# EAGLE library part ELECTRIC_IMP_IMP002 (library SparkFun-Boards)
Electric Imp Module imp002 Datasheet SparkFun Products SparkFun Electric Imp imp002 Breakout (BOB-12958)
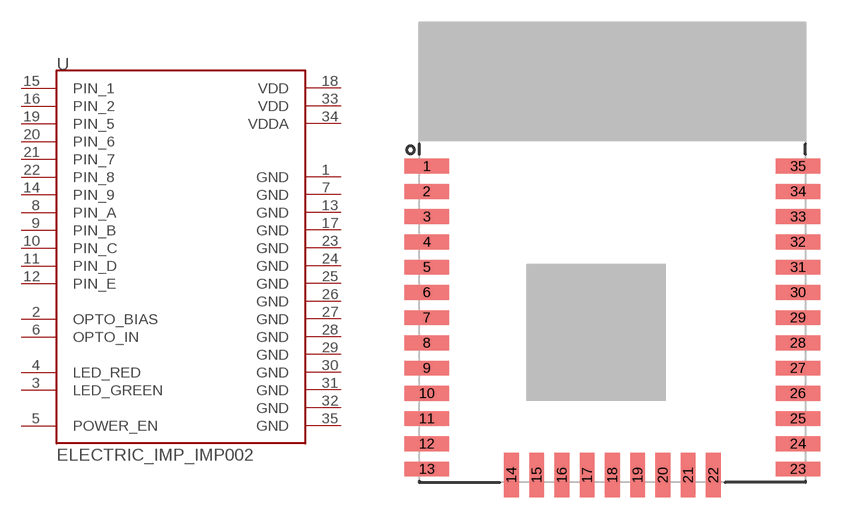
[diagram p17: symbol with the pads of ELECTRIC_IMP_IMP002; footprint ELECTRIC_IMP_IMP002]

Designator prefix U

## ELECTRIC_IMP_IMP002 (PROD_ID: IC-12130; VALUE: imp002)  [ELECTRIC_IMP_IMP002]
1  GND
2  OPTO_BIAS
3  LED_GREEN
4  LED_RED
5  POWER_EN
6  OPTO_IN
7  GND
8  PIN_A
9  PIN_B
10  PIN_C
11  PIN_D
12  PIN_E
13  GND
14  PIN_9
15  PIN_1
16  PIN_2
17  GND
18  VDD
19  PIN_5
20  PIN_6
21  PIN_7
22  PIN_8
23  GND
24  GND
25  GND
26  GND
27  GND
28  GND
29  GND
30  GND
31  GND
32  GND
33  VDD
34  VDDA
35  GND

## Footprint ELECTRIC_IMP_IMP002 (pad centres in mm)
smd 3 x 1: 1 -12.5,5.8; 2 -12.5,4.1; 3 -12.5,2.4; 4 -12.5,0.7; 5 -12.5,-1; 6 -12.5,-2.7; 7 -12.5,-4.4; 8 -12.5,-6.1; 9 -12.5,-7.8; 10 -12.5,-9.5; 11 -12.5,-11.2; 12 -12.5,-12.9; 13 -12.5,-14.6; 23 12.5,-14.6; 24 12.5,-12.9; 25 12.5,-11.2; 26 12.5,-9.5; 27 12.5,-7.8; 28 12.5,-6.1; 29 12.5,-4.4; 30 12.5,-2.7; 31 12.5,-1; 32 12.5,0.7; 33 12.5,2.4; 34 12.5,4.1; 35 12.5,5.8
smd 1 x 3: 14 -6.8,-15; 15 -5.1,-15; 16 -3.4,-15; 17 -1.7,-15; 18 0,-15; 19 1.7,-15; 20 3.4,-15; 21 5.1,-15; 22 6.8,-15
